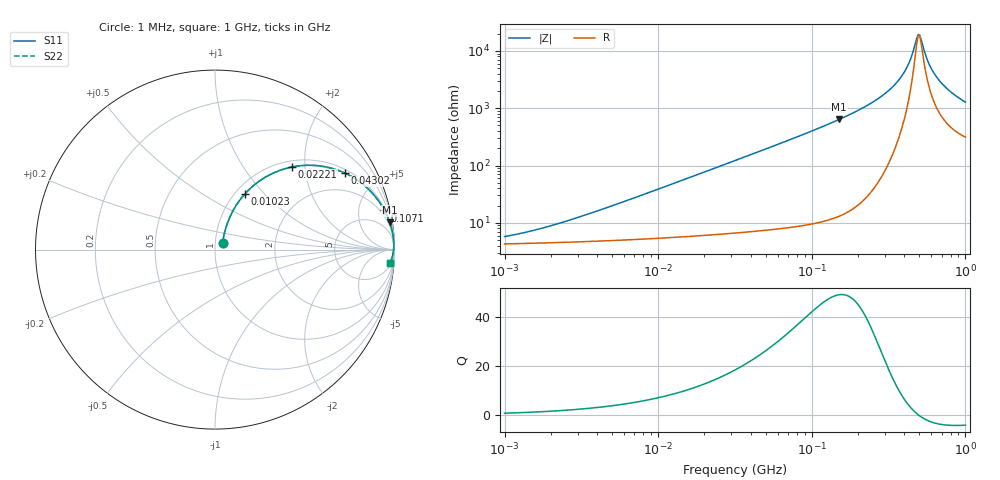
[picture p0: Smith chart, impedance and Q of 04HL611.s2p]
! Coilcraft 0402HL-611 Chip Inductor
! 20 July 2012
# MHz S MA R 50
!Freq  MagS11  AngS11  MagS21  AngS21  MagS12  AngS12  MagS22  AngS22
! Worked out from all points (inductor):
!   304 points, 1 MHz to 1 GHz, reference 50 ohm
!   read as one part in series: L = 610 nH near 3.752 MHz
!   highest Q = 48.9 at 150.7 MHz (marker M1), where L = 672 nH
!   self-resonance near 493.3 MHz
!   S11 on the Smith chart (normalised r, x): 1 MHz: 1.09, +0.08; 10.23 MHz: 1.11, +0.78; 22.21 MHz: 1.12, +1.71; 43.02 MHz: 1.14, +3.32; 107.1 MHz: 1.20, +8.61; 1 GHz: 7, -25
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1  0.05506 39.7  0.9583 -2.1  0.9583 -2.1  0.05506 39.7
3.19853  0.1245 62.4  0.9489 -6.7  0.9489 -6.7  0.1245 62.4
10  0.3453 62.0  0.8919 -20.0  0.8919 -20.0  0.3453 62.0
10.2306  0.3521 61.8  0.8893 -20.4  0.8893 -20.4  0.3521 61.8
22.20929  0.628 47.1  0.7344 -38.8  0.7344 -38.8  0.628 47.1
31.9853  0.7569 37.8  0.614 -49.1  0.614 -49.1  0.7569 37.8
43.0193  0.8412 30.4  0.5059 -57.2  0.5059 -57.2  0.8412 30.4
64.8457  0.9201 21.3  0.3637 -66.9  0.3637 -66.9  0.9201 21.3
102.306  0.9662 13.6  0.2359 -75.0  0.2359 -75.0  0.9662 13.6
107.0787  0.9692 13.0  0.2251 -75.7  0.2251 -75.7  0.9692 13.0
150.7363  0.9848 8.9  0.1548 -79.9  0.1548 -79.9  0.9848 8.9
237.8141  0.9942 4.8  0.08417 -83.6  0.08417 -83.6  0.9942 4.8
319.853  0.9962 2.7  0.0478 -84.1  0.0478 -84.1  0.9962 2.7
366.7384  0.9963 1.9  0.03263 -82.6  0.03263 -82.6  0.9963 1.9
411.0185  0.9961 1.2  0.02059 -78.5  0.02059 -78.5  0.9961 1.2
440.1132  0.9958 0.7  0.0137 -71.8  0.0137 -71.8  0.9958 0.7
493.2525  0.995 0.1  0.005144 -14.0  0.005144 -14.0  0.995 0.1
504.6268  0.9948 -0.1  0.00531 11.9  0.00531 11.9  0.9948 -0.1
578.5971  0.9932 -0.9  0.01658 65.4  0.01658 65.4  0.9932 -0.9
648.457  0.9914 -1.5  0.02823 71.5  0.02823 71.5  0.9914 -1.5
778.1962  0.9873 -2.7  0.04776 73.2  0.04776 73.2  0.9873 -2.7
1000  0.9785 -4.3  0.07657 71.6  0.07657 71.6  0.9785 -4.3
